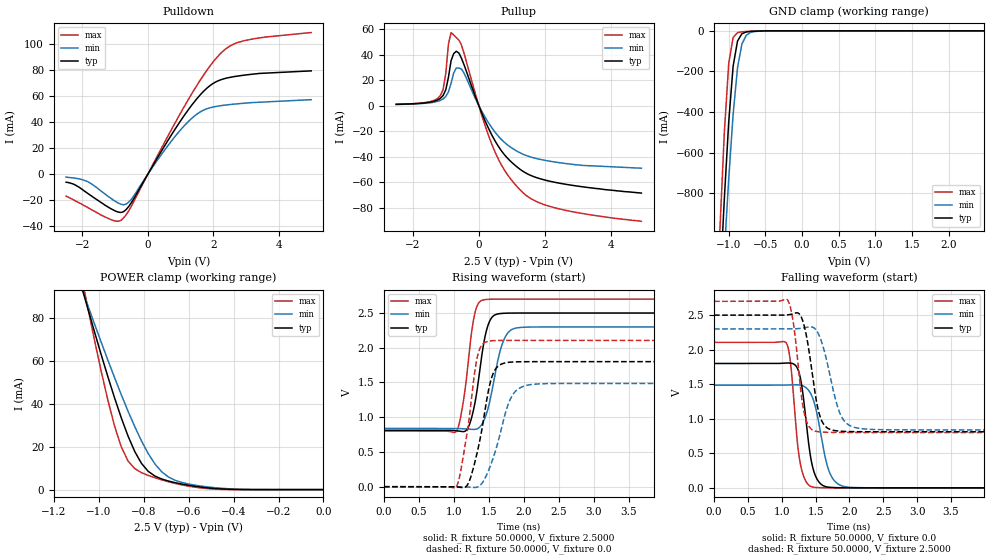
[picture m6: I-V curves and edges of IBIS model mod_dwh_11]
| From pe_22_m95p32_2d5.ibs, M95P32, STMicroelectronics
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|   Model mod_dwh_11
[Model]   mod_dwh_11
Model_type I/O
Polarity   Non-Inverting
Enable   Active-High
Vinl   =   0.750V
Vinh   =   1.750V
Vmeas  =   1.250V
Cref   =   30.0pF
C_comp   1.219pF   1.164pF   1.337pF
[Model Spec]
Vinl   0.750V  0.690V  0.810V  | <- for Vcc = 2.5V, 2.3V, 2.7V
Vinh   1.750V  1.610V  1.890V  | <- for Vcc = 2.5V, 2.3V, 2.7V
Vmeas  1.250V  1.150V  1.350V  | <- for Vcc = 2.5V, 2.3V, 2.7V
[Temperature Range]  25.0000   0.1050k   -40.0000
[Voltage Range]   2.5000V   2.3000V   2.7000V
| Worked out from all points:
|   slope of the pulldown table from 0 to 0.375 V, typ, clamps not added: 23.4 ohm
|   slope of the pullup table from 0 to 0.375 V, typ, clamps not added: 16.9 ohm
|   GND clamp passes 1 mA (typ) near -0.58 V on its own axis
|   POWER clamp passes 1 mA (typ) near -0.53 V on its own axis
|   rising waveform, R_fixture 50.0000, V_fixture 2.5000: 20-80 % time 156ps typ, 187ps min, 139ps max; typ from 0.812 V to 2.5 V
|   rising waveform, R_fixture 50.0000, V_fixture 0.0: 20-80 % time 205ps typ, 257ps min, 172ps max; typ from 0 V to 1.8 V
|   falling waveform, R_fixture 50.0000, V_fixture 0.0: 20-80 % time 141ps typ, 187ps min, 119ps max; typ from 1.8 V to 0 V
|   falling waveform, R_fixture 50.0000, V_fixture 2.5000: 20-80 % time 162ps typ, 218ps min, 132ps max; typ from 2.5 V to 0.812 V
[Pulldown]
|Voltage   I(typ)   I(min)   I(max)
-2.5V     -6.1mA     -2.16mA    -16.8mA
-1.86V    -14.3mA    -5.4mA     -25.2mA
-1.14V    -26.3mA    -18.3mA    -34.7mA
-820mV    -29.37mA   -23.05mA   -35.38mA
-660mV    -27.05mA   -22.93mA   -30.99mA
-500mV    -21.73mA   -19.06mA   -24.39mA
540mV     22.88mA    19.46mA    25.84mA
1.26V     50.29mA    41.01mA    58.29mA
1.74V     64.59mA    49.68mA    77.47mA
2.22V     72.5mA     52.68mA    92.69mA
2.94V     76.14mA    54.59mA    102.6mA
5V        79.45mA    57.32mA    108.9mA
[Pullup]
|Voltage   I(typ)   I(min)   I(max)
-2.5V     960uA      860uA      1.01mA
-1.16V    5.71mA     4.1mA      7.9mA
-1V       12.31mA    7.124mA    25.18mA
-920mV    22.01mA    10.66mA    47.97mA
-840mV    35.12mA    17.46mA    57.19mA
-680mV    42.55mA    29.43mA    53.34mA
-520mV    36.76mA    28.49mA    47.15mA
440mV     -25.32mA   -19.07mA   -33.28mA
840mV     -40.44mA   -30.28mA   -53.17mA
1.32V     -51.25mA   -37.92mA   -67.9mA
2.36V     -60.43mA   -44.46mA   -80.5mA
4.92V     -68.6mA    -49.1mA    -90.7mA
[GND_clamp]
|Voltage   I(typ)   I(min)   I(max)
-2.5V     -12.69A    -11.53A    -14.4A
-1.12V    -1.259A    -1.484A    -977mA
-1.06V    -828.4mA   -1.093A    -501.9mA
-1V       -448.3mA   -729mA     -159.9mA
-940mV    -174mA     -412mA     -32.51mA
-880mV    -50.2mA    -181.6mA   -8.897mA
-820mV    -14.26mA   -64.74mA   -4.945mA
-760mV    -5.535mA   -21.85mA   -3.213mA
-700mV    -3.068mA   -7.635mA   -1.989mA
-640mV    -1.821mA   -3.347mA   -1.073mA
-340mV    -4.191uA   -40.02uA   -134.6nA
2.48V     343.3pA    931.5nA    131.5pA
[POWER_clamp]
|Voltage   I(typ)   I(min)   I(max)
-2.49V    667.2mA    541mA      921mA
-1.08V    96.07mA    95.11mA    101.2mA
-1.05V    84.91mA    86.28mA    85.45mA
-990mV    63.23mA    68.98mA    55.57mA
-930mV    42.88mA    52.31mA    29.76mA
-900mV    33.53mA    44.31mA    19.96mA
-840mV    17.8mA     29.4mA     9.816mA
-810mV    12.22mA    22.72mA    7.905mA
-750mV    6.305mA    11.96mA    5.516mA
-660mV    3.226mA    4.34mA     2.89mA
-420mV    154.8uA    392.4uA    29.01uA
0V        492.2pA    14.11nA    240.5pA
[Ramp]
| variable   typ   min   max
dV/dt_r  1.0800/0.2734n   0.9088/0.3125n   1.2634/0.2481n
dV/dt_f  1.0131/0.2548n   0.8870/0.2879n   1.1391/0.2416n
R_load = 50.0000
[Rising Waveform]
R_fixture= 50.0000
V_fixture= 2.5000
V_fixture_min= 2.3000
V_fixture_max= 2.7000
|time   V(typ)   V(min)   V(max)
0s        811.6mV    838.9mV    801.5mV
1.032ns   805.5mV    838.8mV    791.4mV
1.136ns   792.6mV    833.7mV    1.232V
1.24ns    946.3mV    825.7mV    2.12V
1.32ns    1.314V     828.4mV    2.569V
1.432ns   2.093V     959.8mV    2.691V
1.528ns   2.415V     1.297V     2.699V
1.688ns   2.495V     2.043V     2.7V
1.896ns   2.5V       2.285V     2.7V
8ns       2.5V       2.3V       2.7V
[Rising Waveform]
R_fixture= 50.0000
V_fixture= 0.0
V_fixture_min= 0.0
V_fixture_max= 0.0
|time   V(typ)   V(min)   V(max)
0s        3.45nV     419.9nV    574.2pV
1.024ns   -2.38mV    831.1uV    -11.17mV
1.096ns   -9.776mV   -3.697uV   217.3mV
1.24ns    135.2mV    -7.605mV   1.162V
1.352ns   575.4mV    1.858mV    1.935V
1.48ns    1.31V      196.2mV    2.091V
1.592ns   1.688V     506.4mV    2.104V
1.8ns     1.792V     1.244V     2.106V
2.056ns   1.8V       1.462V     2.106V
8ns       1.8V       1.486V     2.106V
[Falling Waveform]
R_fixture= 50.0000
V_fixture= 0.0
V_fixture_min= 0.0
V_fixture_max= 0.0
|time   V(typ)   V(min)   V(max)
0s        1.8V       1.486V     2.106V
1.064ns   1.807V     1.488V     2.101V
1.128ns   1.805V     1.491V     1.823V
1.224ns   1.745V     1.493V     720.8mV
1.272ns   1.603V     1.487V     361.8mV
1.448ns   334.1mV    1.322V     13.96mV
1.544ns   91.4mV     959.1mV    3.748mV
1.688ns   9.787mV    270.8mV    674.4uV
1.928ns   1.005mV    17.9mV     42.02uV
8ns       962.7nV    1.54uV     983.6nV
[Falling Waveform]
R_fixture= 50.0000
V_fixture= 2.5000
V_fixture_min= 2.3000
V_fixture_max= 2.7000
|time   V(typ)   V(min)   V(max)
0s        2.5V       2.3V       2.7V
1.088ns   2.504V     2.299V     2.717V
1.176ns   2.523V     2.301V     2.356V
1.304ns   2.434V     2.312V     1.234V
1.384ns   2.095V     2.327V     920.6mV
1.496ns   1.347V     2.298V     820.1mV
1.608ns   938mV      2.053V     806.5mV
1.848ns   821.6mV    1.107V     801.8mV
2.088ns   812.9mV    872mV      801.5mV
8ns       811.6mV    838.9mV    801.5mV
